FUNCTION_BLOCK NullSubstate EXTENDS Substate
VAR
END_VAR

METHOD PUBLIC IsEqual : BOOL
VAR_INPUT
	Substate : I_Substate;
END_VAR
IsEqual := false;
END_METHOD

PROPERTY PUBLIC Name : T_MAXSTRING
GET
Name := '';
END_GET
END_PROPERTY

END_FUNCTION_BLOCK
